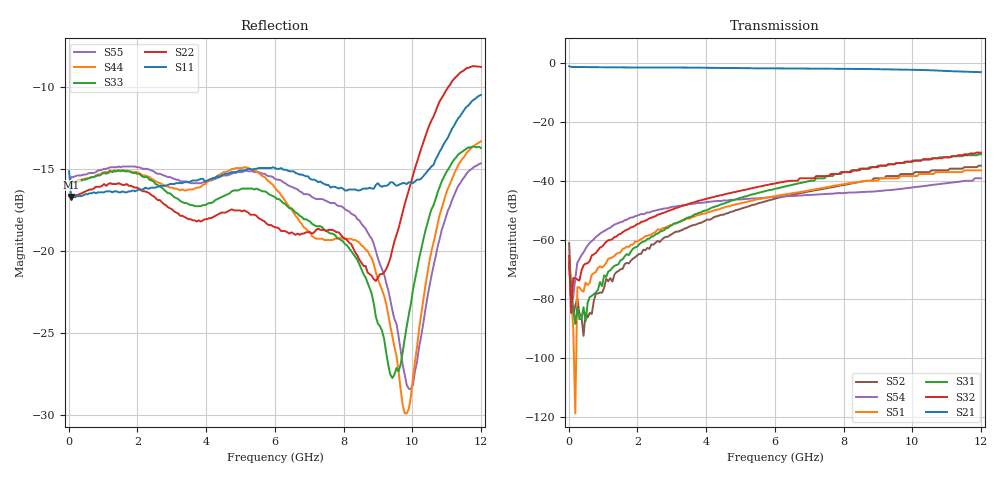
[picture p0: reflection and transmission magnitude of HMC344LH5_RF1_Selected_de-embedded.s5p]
! Hittite Microwave Corporation
! 20 Alpha Road
! Chelmsford, MA 01824
! Tel: 978-250-3343
! Fax: 978-250-3373
! Device: HMC344LH5, DC-12 GHz GaAs MMIC SP4T Non-Reflective Switch in Hermetic Leadless SMT Package
! Misc: Data was de-embedded to package pins.
!  Port 1 = RFC
!  Port 2 = RF1
!  Port 3 = RF2
!  Port 4 = RF3
!  Port 5 = RF4
!  RF1 selected, Vctl= 0/-5 V
!  Data reformated to new Touchstone file format - Tue Jan 09 13:12:26 2007
# MHz S DB R 50
! 5 Port Network Data
! freq  dbS11  angS11  dbS12  angS12  dbS13  angS13  dbS14  angS14
!  dbS15  angS15
!  dbS21  angS21  dbS22  angS22  dbS23  angS23
!  dbS24  angS24  dbS25  angS25
!  dbS31  angS31  dbS32  angS32
!  dbS33  angS33  dbS34  angS34  dbS35  angS35
!  dbS41  angS41
!  dbS42  angS42  dbS43  angS43  dbS44  angS44  dbS45  angS45
!  dbS51  angS51  dbS52  angS52  dbS53  angS53  dbS54  angS54
!  dbS55  angS55
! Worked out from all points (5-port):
!   201 points, 10 MHz to 12 GHz, reference 50 ohm
!   strongest paths, dB at 10 MHz, 3.007 GHz, 6.005 GHz, 9.002 GHz, 12 GHz:
!     S21: -1.2, -1.7, -2.0, -2.3, -3.3
!     S32: -65.3, -49.7, -40.9, -35.4, -30.5
!     S31: -67.3, -55.0, -42.7, -34.9, -31.1
!     S51: -68.9, -54.8, -45.2, -40.0, -36.5
!     S54: -67.6, -48.8, -45.5, -43.5, -39.2
!     S52: -61.1, -58.0, -46.1, -39.2, -34.9
!   lowest |S11| = -16.7 dB at 69.95 MHz (marker M1), VSWR 1.34, Z = 67.1 - j0.836 ohm
!   |S11| at or under -10 dB: start of sweep to end of sweep
